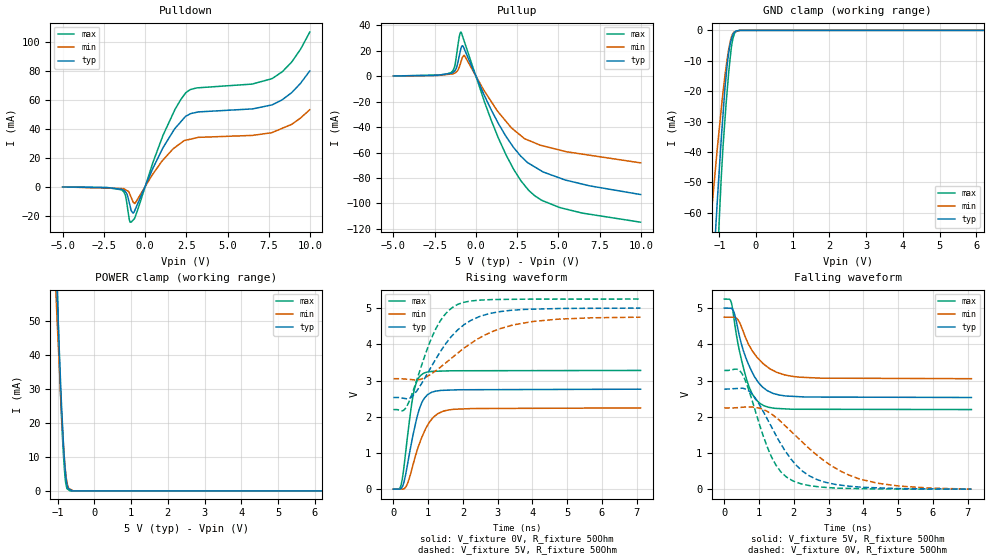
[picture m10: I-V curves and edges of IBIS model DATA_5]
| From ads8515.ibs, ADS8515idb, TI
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|   DATA OUTPUT Model  5V
[Model] DATA_5
Model_type 3-state
Polarity   Non-Inverting
Enable   Active-Low
Vmeas = 2.5
Vref = 2.5
Cref = 15pF
Rref = 50
|   typ   min   max
| AVERAGE
C_comp   8.4321450E-12   8.4233490E-12   9.3228145E-12
| HIGH out
|C_comp   9.2103230e-12   8.3870010e-12   1.0168340e-11
| LOW out
|C_comp   8.4772890e-12   7.6363750e-12   8.4772890e-12
[Voltage Range]   5   4.75   5.25
[Temperature Range]   27   85   -40
[Pullup Reference]   5   4.75   5.25
[Pulldown Reference]   0   0   0
[Power Clamp Reference]   5   4.75   5.25
[GND Clamp Reference]   0   0   0
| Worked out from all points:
|   slope of the pulldown table from 0 to 0.75 V, typ, clamps not added: 39.4 ohm
|   slope of the pullup table from 0 to 0.75 V, typ, clamps not added: 34.4 ohm
|   GND clamp passes 1 mA (typ) near -0.61 V on its own axis
|   POWER clamp passes 1 mA (typ) near -0.72 V on its own axis
|   falling waveform, V_fixture 5V, R_fixture 50Ohm: 20-80 % time 551ps typ, 698ps min, 431ps max; typ from 5 V to 2.53 V
|   rising waveform, V_fixture 0V, R_fixture 50Ohm: 20-80 % time 365ps typ, 500ps min, 266ps max; typ from 0 V to 2.76 V
|   rising waveform, V_fixture 5V, R_fixture 50Ohm: 20-80 % time 1.11ns typ, 1.63ns min, 744ps max; typ from 2.53 V to 5 V
|   falling waveform, V_fixture 0V, R_fixture 50Ohm: 20-80 % time 1.11ns typ, 1.75ns min, 748ps max; typ from 2.76 V to 0 V
[Pulldown]
|   Voltage   I  typ   I  min   I  max
-5V       -196.9uA   -156.9uA   -196.2uA
-1.437V   -1.791mA   -1.283mA   -2.151mA
-1.198V   -3.427mA   -2.049mA   -5.886mA
-960.5mV  -11.01mA   -4.199mA   -22.8mA
-847.1mV  -16.34mA   -7.323mA   -24.6mA
-592.6mV  -15.6mA    -11.28mA   -20.57mA
1.101V    27.32mA    18.7mA     36mA
1.808V    40.32mA    27.18mA    53.45mA
2.461V    48.78mA    32.18mA    65.01mA
7.665V    56.63mA    37.4mA     74.79mA
8.859V    64.93mA    43.08mA    86.02mA
9.985V    80.24mA    53.37mA    107.2mA
[GND Clamp]
|   Voltage   I  typ   I  min   I  max
-5V       -1.015A    -749.1mA   -1.377A
-1.237V   -94.64mA   -63.73mA   -133.2mA
-1.153V   -76.63mA   -52.16mA   -106.9mA
-1.071V   -59.86mA   -41.17mA   -82.26mA
-1.022V   -50.14mA   -35.14mA   -68.45mA
-1.003V   -46.62mA   -32.87mA   -63.12mA
-943.6mV  -35.46mA   -25.7mA    -48.03mA
-892.1mV  -26.81mA   -19.77mA   -37.37mA
-778.3mV  -10.63mA   -8.974mA   -19.01mA
-661.1mV  -2.466mA   -2mA       -4.898mA
-549.6mV  -247.9uA   -411.1uA   -491.3uA
9.985V    0A         0A         0A
[Pullup]
|   Voltage   I  typ   I  min   I  max
-5V       265.1uA    227.5uA    280.9uA
-1.511V   2.335mA    1.741mA    2.969mA
-1.287V   4.114mA    2.556mA    7.784mA
-1.009V   16mA       7.184mA    31.17mA
-908.3mV  21.94mA    11.3mA     34.81mA
-808.9mV  24.08mA    15.12mA    31.53mA
-681.5mV  20.79mA    16.1mA     26.57mA
1.381V    -37.58mA   -28.52mA   -49.12mA
2.309V    -56.39mA   -42.25mA   -73.65mA
3.187V    -68.33mA   -50.37mA   -89.54mA
5.074V    -80mA      -58.03mA   -103.2mA
9.985V    -93.04mA   -68.11mA   -114.8mA
[POWER Clamp]
|   Voltage   I  typ   I  min   I  max
-5V       1.738A     1.463A     2.143A
-1.047V   69.57mA    58.51mA    75.94mA
-1.009V   57.33mA    48.99mA    59.45mA
-1.003V   55.65mA    47.72mA    57.17mA
-960.5mV  42.82mA    37.94mA    40.81mA
-920.6mV  32.17mA    28.84mA    28.23mA
-837mV    12.9mA     12.71mA    9.845mA
-796.9mV  6.725mA    7.14mA     4.024mA
-761.2mV  2.923mA    3.512mA    1.361mA
-717mV    765.5uA    1.283mA    455.7uA
-661.1mV  395.3uA    536.2uA    12.3uA
9.985V    0A         0A         0A
[Ramp]
R_load = 50
|   typ   min   max
dV/dt_r   1.65662/3.6426e-010   1.34625/4.96781e-010   1.96737/2.65374e-010
dV/dt_f   1.48099/5.4782e-010   1.01944/6.87753e-010   1.83103/4.30221e-010
[Falling Waveform]
V_fixture = 5V
V_fixture_min = 4.75V
V_fixture_max = 5.25V
R_fixture = 50Ohm
C_fixture = 0F
|   Time   V  typ   V  min   V  max
0s        5V         4.75V      5.25V
201.6ps   4.994V     4.75V      5.158V
291.4ps   4.851V     4.748V     4.629V
427.1ps   4.263V     4.626V     3.862V
709.7ps   3.421V     3.982V     2.835V
893.3ps   3.072V     3.705V     2.493V
1.134ns   2.795V     3.455V     2.308V
1.504ns   2.619V     3.229V     2.23V
2.163ns   2.554V     3.093V     2.207V
7.11ns    2.532V     3.051V     2.198V
[Rising Waveform]
V_fixture = 0V
V_fixture_min = 0V
V_fixture_max = 0V
R_fixture = 50Ohm
C_fixture = 0F
|   Time   V  typ   V  min   V  max
0s        -1.551uV   -3.55uV    -2.015uV
220.2ps   19.05mV    713.3uV    116mV
362.6ps   466.2mV    69.45mV    1.112V
477.2ps   1.074V     369.4mV    2.024V
574.8ps   1.547V     715.9mV    2.632V
697.1ps   2.056V     1.122V     3.026V
868.8ps   2.48V      1.546V     3.202V
1.274ns   2.715V     2.084V     3.258V
1.73ns    2.74V      2.205V     3.27V
7.11ns    2.761V     2.244V     3.279V
[Rising Waveform]
V_fixture = 5V
V_fixture_min = 4.75V
V_fixture_max = 5.25V
R_fixture = 50Ohm
C_fixture = 0F
|   Time   V  typ   V  min   V  max
0s        2.532V     3.051V     2.198V
361.5ps   2.499V     3.039V     2.248V
659.6ps   2.696V     3.014V     2.982V
1.209ns   3.579V     3.264V     4.411V
1.513ns   4.029V     3.495V     4.858V
1.85ns    4.4V       3.758V     5.103V
2.495ns   4.775V     4.186V     5.222V
3.46ns    4.944V     4.538V     5.243V
4.756ns   4.989V     4.696V     5.249V
7.11ns    5V         4.75V      5.25V
[Falling Waveform]
|Gnd
V_fixture = 0V
V_fixture_min = 0V
V_fixture_max = 0V
R_fixture = 50Ohm
C_fixture = 0F
|   Time   V  typ   V  min   V  max
0s        2.761V     2.244V     3.279V
508.7ps   2.788V     2.261V     3.194V
870.5ps   2.545V     2.26V      2.233V
1.356ns   1.725V     2.076V     897.4mV
1.629ns   1.249V     1.864V     478.2mV
1.966ns   778.6mV    1.556V     233mV
2.666ns   266mV      940.4mV    71.15mV
3.874ns   60.05mV    287.8mV    15.39mV
5.053ns   15.81mV    84.17mV    4.026mV
7.11ns    -1.551uV   -3.55uV    -2.015uV
